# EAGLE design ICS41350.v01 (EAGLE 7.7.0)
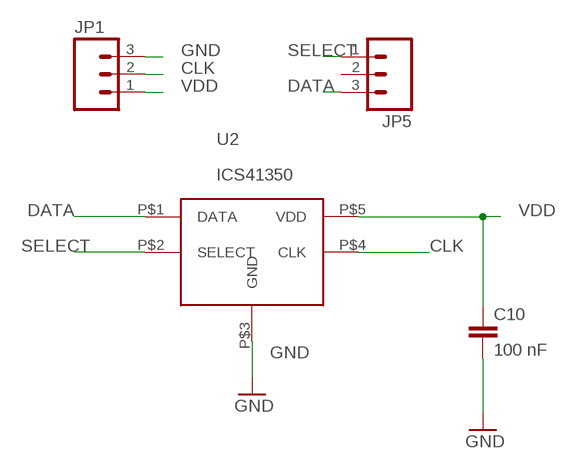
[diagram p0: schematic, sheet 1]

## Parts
C10  100 nF  0402CAP.KW  [0402-CAP]
JP1  M031X03_NO_SILK  [1X03_NO_SILK]
JP5  M031X03_NO_SILK  [1X03_NO_SILK]
U2  ICS41350  [ICS41350]

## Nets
CLK: JP1.2 U2.P$4(CLK)
DATA: JP5.3 U2.P$1(DATA)
GND: C10.2 JP1.3 U2.P$3(GND)
SELECT: JP5.1 U2.P$2(SELECT)
VDD: C10.1 JP1.1 U2.P$5(VDD)
Unconnected: JP5.2

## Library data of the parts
C10 = SparkFun-Capacitors:0402CAP.KW
JP1 JP5 = SparkFun-Connectors:M03: Header 3 Standard 3-pin 0.1" header. Use with straight break away headers (SKU : PRT-00116), right angle break away headers (PRT-00553), swiss pins (PRT-00743), machine pins (PRT-00117), and female headers (PRT-00115). Molex polarized connector foot print use with SKU : PRT-08232 with associated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
U2 = kris:ICS41350: Invensense's ICS4135X PDM microphone

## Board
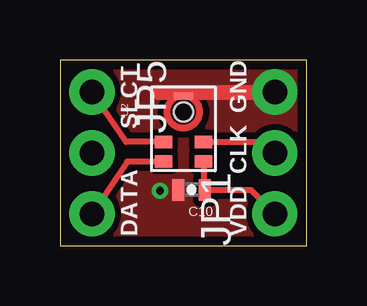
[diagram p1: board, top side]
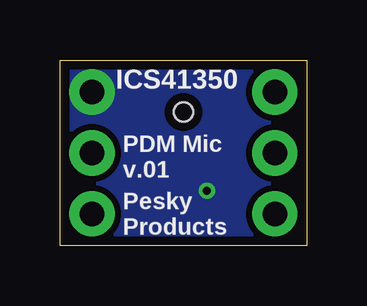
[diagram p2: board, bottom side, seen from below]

Size 10.29 x 7.75 mm. Coordinates in mm from the lower left corner, seen from the top.
Outline: 0,0 10.29,0 10.29,7.75 0,7.75 0,0
Copper layers (1*16): Top 0.0356mm / dielectric 1.5011mm / Bottom 0.0356mm
Design rules "LaenPCBOrder *": minimum track width 6mil, minimum drill 13mil, track to track 6mil, track to pad 6mil, pad to pad 6mil, via to via 6mil, smd to smd 6mil, copper to edge 15mil, drill to drill 6mil, minimum pad ring 7mil, minimum via ring 7mil, stop-mask expansion 3mil, vias tented up to drill 20mil, thermal gap 10mil

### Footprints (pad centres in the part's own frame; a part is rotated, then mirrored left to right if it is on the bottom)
0402-CAP = smd 0.5 x 0.9: 1 -0.55,0; 2 0.55,0
1X03_NO_SILK = drill 1.016 pad 1.88: 1 0,0; 2 2.54,0; 3 5.08,0
ICS41350 = smd 0.522 x 0.725: P$1 -1.364,0.838; P$2 -0.542,0.838; P$4 -0.542,-0.838; P$5 -1.364,-0.838 | smd 0.3 x 0.8: P$3 1.37,0 | hole 0.8: 0.71,0

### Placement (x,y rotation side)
C10  5.49,2.34 180 top
JP1  8.95,1.33 90 top
JP5  1.33,6.41 270 top
U2  5.14,4.88 90 top

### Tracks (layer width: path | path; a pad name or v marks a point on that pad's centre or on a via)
CLK
  Top 0.254: U2.P$4 8.49,4.33 JP1.2
DATA
  Top 0.254: U2.P$1 2.8,3.51 JP5.3
GND  (via drill 0.33)
  Top 0.305: JP1.3 8.81,6.55 3.96,6.55 3.96,6.35 4.07,6.25 U2.P$3 8.63,6.25 8.89,6.5
  other vias: 4.17,2.3
  pour Bottom (isolate 0.254, no thermals): 0,7.75 10.29,7.75 10.29,0 0,0
  pour Top (isolate 0.254, no thermals): 0,7.75 10.29,7.75 10.29,0 0,0
SELECT
  Top 0.254: U2.P$2 2.75,4.33 JP5.1
VDD
  Top 0.254: U2.P$5 5.98,2.39 C10.1 7.95,2.34 JP1.1

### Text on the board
tPlace: GND | SLCT | CLK | DATA | VDD
bPlace: ICS41350 | PDM Mic | v.01 | Pesky / Products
